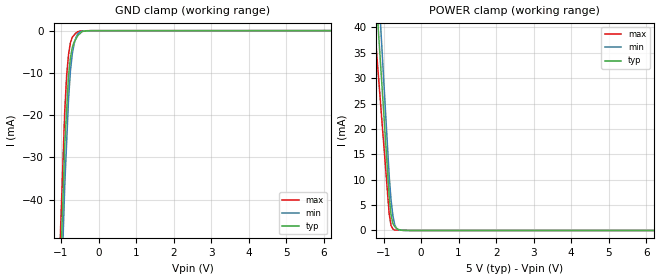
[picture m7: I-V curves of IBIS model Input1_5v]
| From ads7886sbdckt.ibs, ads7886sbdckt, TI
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[Model] Input1_5v
Model_type Terminator
C_comp 1.513pF 1.513pF 1.513pF
| variable typ   min   max
[Voltage Range] 5.00000V 4.75000V 5.25000V
[POWER Clamp Reference] 5.00000V 4.75000V 5.25000V
[GND Clamp Reference] 0.00000V 0.00000V 0.00000V
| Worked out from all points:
|   GND clamp passes 1 mA (typ) near -0.53 V on its own axis
|   POWER clamp passes 1 mA (typ) near -0.72 V on its own axis
[GND Clamp]
-5V       -1.105A    -1.17A     -1.047A
-900mV    -26.98mA   -36.4mA    -18.85mA
-850mV    -18.78mA   -26.31mA   -10.63mA
-800mV    -10.59mA   -16.22mA   -5.654mA
-750mV    -6.448mA   -9.596mA   -2.885mA
-700mV    -3.987mA   -5.467mA   -1.558mA
-650mV    -2.686mA   -3.064mA   -1.038mA
-600mV    -1.914mA   -1.538mA   -518.3uA
-550mV    -1.141mA   -731.2uA   -242.9uA
-400mV    -116.9uA   -100.4uA   -54.36uA
-200mV    -7.089uA   -10.34uA   -4.808uA
10V       10.21uA    16.05uA    6.918uA
[POWER Clamp]
-5V       477.6mA    549.9mA    396.5mA
-1.1V     35.15mA    43.27mA    27mA
-1.05V    29.47mA    36.78mA    22.26mA
-850mV    6.781mA    10.8mA     3.316mA
-800mV    3.069mA    5.987mA    980.4uA
-750mV    1.376mA    2.87mA     277.5uA
-700mV    743uA      1.087mA    81.07uA
-650mV    408.2uA    376.9uA    72.53uA
-600mV    189.6uA    120.5uA    64uA
-400mV    11.04uA    0A         29.87uA
10V       0A         0A         0A
